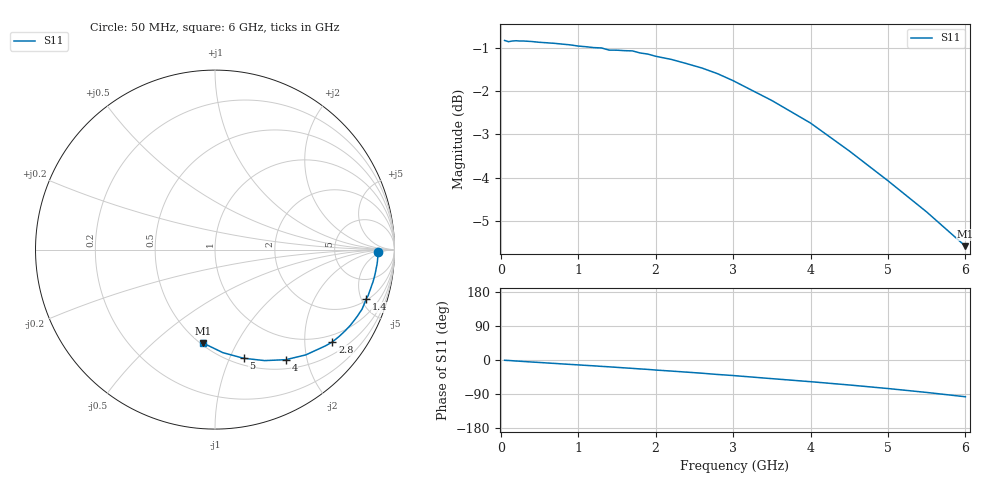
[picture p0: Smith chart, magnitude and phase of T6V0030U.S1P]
! SIEMENS Discrete & RF Semiconductors
! BAT62
! Si Schottky Diode in SOT143
! IF = 0.03 mA
! S-Parameters:  February  1997
# GHz  S  MA  R  50
!  f  S11
! GHz  MAG  ANG
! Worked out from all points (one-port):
!   34 points, 50 MHz to 6 GHz, reference 50 ohm
!   lowest |S11| = -5.6 dB at 6 GHz (marker M1), VSWR 3.22, Z = 25.8 - j37.2 ohm
!   |S11| at or under -10 dB: nowhere
!   S11 on the Smith chart (normalised r, x): 50 MHz: 21, -3; 1.4 GHz: 2.16, -5.49; 2.8 GHz: 0.80, -2.68; 4 GHz: 0.63, -1.65; 5 GHz: 0.57, -1.13; 6 GHz: 0.52, -0.74
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0.05  0.9089 -0.7
0.1  0.9059 -1.3
0.15  0.9075 -1.9
0.2  0.9081 -2.7
0.4  0.9063 -5.3
0.5  0.9044 -6.5
0.7  0.9018 -9.1
0.8  0.9 -10.4
0.9  0.8982 -11.7
1.2  0.8918 -15.4
1.3  0.891 -16.8
1.4  0.8858 -18.0
1.6  0.8845 -20.8
1.7  0.884 -22.1
1.8  0.8791 -23.6
1.9  0.8765 -24.8
2  0.8714 -26.5
2.2  0.8642 -29.2
2.4  0.8546 -32.0
2.6  0.8445 -34.9
2.8  0.8319 -38.2
3  0.8167 -41.0
3.5  0.7748 -49.2
4  0.7296 -57.2
4.5  0.6775 -65.9
5  0.6258 -75.3
5.5  0.5759 -85.6
6  0.5258 -97.0
